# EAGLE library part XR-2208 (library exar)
Operational MULTIPLIER
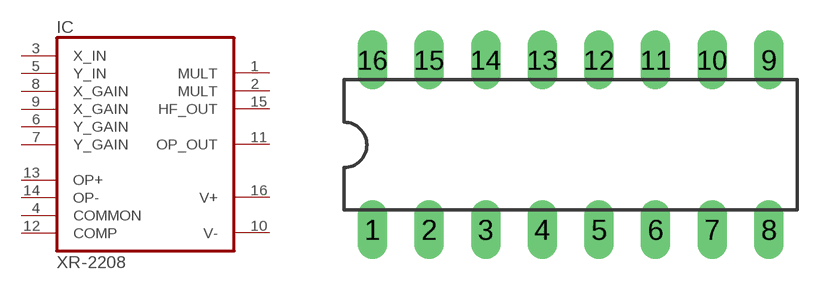
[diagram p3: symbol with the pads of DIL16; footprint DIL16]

Designator prefix IC

## XR-2208 (OC_FARNELL: unknown; OC_NEWARK: unknown)  [DIL16]
1  MULT  out
2  MULT  out
3  X_IN  in
4  COMMON  in
5  Y_IN  in
6  Y_GAIN  in
7  Y_GAIN  in
8  X_GAIN  in
9  X_GAIN  in
10  V-  pwr
11  OP_OUT  out
12  COMP  in
13  OP+  in
14  OP-  in
15  HF_OUT  out
16  V+  pwr

## Footprint DIL16 (pad centres in mm)
Dual In Line Package
drill 0.813 long: 1 -8.89,-3.81; 2 -6.35,-3.81; 3 -3.81,-3.81; 4 -1.27,-3.81; 5 1.27,-3.81; 6 3.81,-3.81; 7 6.35,-3.81; 8 8.89,-3.81; 9 8.89,3.81; 10 6.35,3.81; 11 3.81,3.81; 12 1.27,3.81; 13 -1.27,3.81; 14 -3.81,3.81; 15 -6.35,3.81; 16 -8.89,3.81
